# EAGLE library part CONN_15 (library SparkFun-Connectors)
Multi connection point. Often used as Generic Header-pin footprint for 0.1 inch spaced/style header connections On any of the 0.1 inch spaced packages, you can populate with these: Break Away Headers - Straight (PRT-00116) Break Away Male Headers - Right Angle (PRT-00553) Female Headers (PRT-00115) Break Away Headers - Machine Pin (PRT-00117) Break Away Female Headers - Swiss Machine Pin (PRT-00743) For SCREWTERMINALS and SPRING TERMINALS visit here: Screw Terimnals on SparkFun.com (5mm/3.5mm/2.54mm spacing) This device is also useful as a general connection point to wire up your design to another part of your project. Our various solder wires solder well into these plated through hole pads. Hook-Up Wire - Assortment (Stranded, 22 AWG) (PRT-11375) Hook-Up Wire - Assortment (Solid Core, 22 AWG) (PRT-11367) View the entire wire category on our website here Special notes: Molex polarized connector foot print use with SKU : PRT-08231 with associated crimp pins and housings. 1MM SMD Version SKU: PRT-10208 NOTES ON THE VARIANTS LOCK and LOCK_LONGPADS... This footprint was designed to help hold the alignment of a through-hole component (i.e. 6-pin header) while soldering it into place. You may notice that each hole has been shifted either up or down by 0.005 of an inch from it's more standard position (which is a perfectly straight line). This slight alteration caused the pins (the squares in the middle) to touch the edges of the holes. Because they are alternating, it causes a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
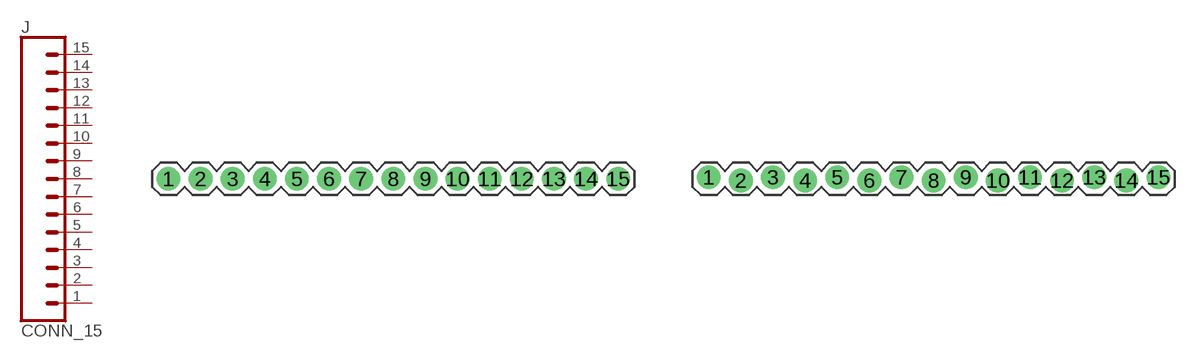
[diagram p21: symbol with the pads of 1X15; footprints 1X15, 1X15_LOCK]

Designator prefix J

## CONN_15  [1X15]
1  1  pas
2  2  pas
3  3  pas
4  4  pas
5  5  pas
6  6  pas
7  7  pas
8  8  pas
9  9  pas
10  10  pas
11  11  pas
12  12  pas
13  13  pas
14  14  pas
15  15  pas

## CONN_15LOCK  [1X15_LOCK]
Pads as for 1X15

## CONN_15LOCK_LONGPADS  [1X15_LOCK_LONGPADS]
Pads as for 1X15

## CONN_15LOCK_NO_SILK  [1X15_LOCK_NO_SILK]
Pads as for 1X15

## Footprint 1X15 (pad centres in mm)
Plated Through Hole -15 Pin Specifications: Pin count:15 Pin pitch:0.1" Example device(s): CONN_15
drill 1.016 pad 1.88: 1 0,0; 2 2.54,0; 3 5.08,0; 4 7.62,0; 5 10.16,0; 6 12.7,0; 7 15.24,0; 8 17.78,0; 9 20.32,0; 10 22.86,0; 11 25.4,0; 12 27.94,0; 13 30.48,0; 14 33.02,0; 15 35.56,0

## Footprint 1X15_LOCK (pad centres in mm)
Plated Through Hole -15 Pin Locking Footprint Holes are offset 0.005" to hold pins in place while soldering. Specifications: Pin count:15 Pin pitch:0.1" Example device(s): CONN_15
drill 1.016 pad 1.88: 1 0,0.127; 2 2.54,-0.127; 3 5.08,0.127; 4 7.62,-0.127; 5 10.16,0.127; 6 12.7,-0.127; 7 15.24,0.127; 8 17.78,-0.127; 9 20.32,0.127; 10 22.86,-0.127; 11 25.4,0.127; 12 27.94,-0.127; 13 30.48,0.127; 14 33.02,-0.127; 15 35.56,0.127

## Footprint 1X15_LOCK_LONGPADS (pad centres in mm)
Plated Through Hole -15 Pin Locking Footprint with Long Pads Holes are offset 0.005" to hold pins in place while soldering. Specifications: Pin count:15 Pin pitch:0.1" Example device(s): CONN_15
drill 1.016 long: 1 0,0.127; 2 2.54,-0.127; 3 5.08,0.127; 4 7.62,-0.127; 5 10.16,0.127; 6 12.7,-0.127; 7 15.24,0.127; 8 17.78,-0.127; 9 20.32,0.127; 10 22.86,-0.127; 11 25.4,0.127; 12 27.94,-0.127; 13 30.48,0.127; 14 33.02,-0.127; 15 35.56,0.127

## Footprint 1X15_LOCK_NO_SILK (pad centres in mm)
Plated Through Hole -15 Pin Locking Footprint No Silk Outline Holes are offset 0.005" to hold pins in place while soldering. Specifications: Pin count:15 Pin pitch:0.1" Example device(s): CONN_15
drill 1.016 pad 1.88: 1 0,0.127; 2 2.54,-0.127; 3 5.08,0.127; 4 7.62,-0.127; 5 10.16,0.127; 6 12.7,-0.127; 7 15.24,0.127; 8 17.78,-0.127; 9 20.32,0.127; 10 22.86,-0.127; 11 25.4,0.127; 12 27.94,-0.127; 13 30.48,0.127; 14 33.02,-0.127; 15 35.56,0.127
